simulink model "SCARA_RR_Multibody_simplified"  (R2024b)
settings: Solver=VariableStepAuto  StartTime=0.0  StopTime=5  RelTol=1e-3  EnableMultiTasking=on
undefined symbols (not defined in the file or in its folder): deg, kg, m, N, s
libraries: sm_lib x11, nesl_utility x9

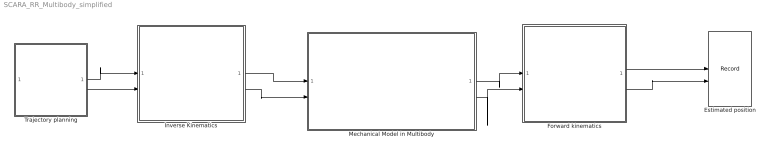
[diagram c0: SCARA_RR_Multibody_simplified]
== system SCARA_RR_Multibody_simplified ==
  Estimated position : Record  FileSettingsInternal="{\"entries\":[{\"content\":{\"excelSettings\":{\"content\":{},\"type\":\"Streamout.ExcelSettings\"}},\"type\":\"Streamout.FileSettingStorage\",\"uuid\":\"\"}],\"packageUris\":[\"http:\\/\\/schema.mathworks.com\\/mf0\\/streamout_blocks\\/R2020a\"],\"version\":\"1.0\"}"  Layout=[1 1]  SignalsInternal="{\"entries\":[{\"content\":{\"signals\":[{\"content\":{\"blockPath\":[],\"dimensions\":[1],\"domain\":\"\",\"lineColor\":\"#ff6929\",\"lineWidth\":2,\"port\":1,\"sid\":[\"\"],\"signalID\":1,\"signalName\":\"Forward kinematics:1\"},\"type\":\"RecordBlkView.Signal\",\"uuid\":\"\"},{\"content\":{\"blockPath\":[],\"dimensions\":[1],\"domain\":\"\",\"lineColor\":\"#b746ff\",\"lineWidth\":2,\"port\":2,\"sid\":[\"\"],\"signalID\":2,\"signalName\":\"Forward kinematics:2\"},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"  VisualizationBindings="{\"xyplotplugin\":{\"info\":[{\"series\":[],\"subplotID\":1}]}}"  CompatibilityTag=XY  st=-1
  Forward kinematics : MATLAB Function  TreatAsAtomicUnit=on
  Inverse Kinematics : MATLAB Function  TreatAsAtomicUnit=on
  Mechanical Model in Multibody : Subsystem
  Trajectory planning : Subsystem
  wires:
  Forward kinematics/2(Y) -> Estimated position/2
  Forward kinematics/1(X) -> Estimated position/1
  Trajectory planning/1(Xd) -> Inverse Kinematics/1(Xd)
  Trajectory planning/2(Yd) -> Inverse Kinematics/2(Yd)
  Inverse Kinematics/1(Theta1) -> Mechanical Model in Multibody/1(Theta1d)
  Inverse Kinematics/2(Theta2) -> Mechanical Model in Multibody/2(Theta 2d)
  Mechanical Model in Multibody/1(Theta1) -> Forward kinematics/1(Theta1)
  Mechanical Model in Multibody/2(Theta2) -> Forward kinematics/2(Theta2)

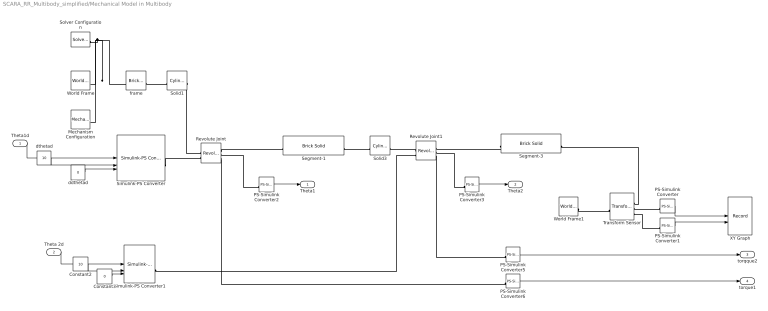
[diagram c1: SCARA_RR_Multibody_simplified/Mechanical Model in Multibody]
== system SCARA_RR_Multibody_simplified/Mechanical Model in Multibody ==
  Theta1d : Inport
  Theta 2d : Inport  Port=2
  Constant2 : Constant  Value=10
  Constant3 : Constant  Value=0
  Mechanism Configuration : sm_lib/Utilities/Mechanism Configuration  UniformGravity=Constant  GravityVector=[0 -9.80665 0]  GravityVectorUnits=m/s^2  LinearizationDelta=0.001  JointModeTransitionNonlinearIterations=2
  PS-Simulink Converter{,1..3,5..6} (6 alike) : nesl_utility/PS-Simulink Converter  PhysicalDomain=network_engine_domain  SubClassName=ps_output  LeftPortType=input  RightPortType=output  PseudoPeriodic=off  Frequencies=[]  VectorFormat=1-D array  Unit=1  AffineConversion=off
  Revolute Joint : sm_lib/Joints/Revolute Joint  JointMode=Normal  CompositeWrenchDir=FollowerOnBase  CompositeWrenchFrame=BaseFrame  SenseConstraintForce=off  SenseConstraintTorque=off  SenseTotalForce=off  SenseTotalTorque=off  PositionTargetSpecify=off  PositionTargetPriority=High  PositionTargetValue=0  PositionTargetValueUnits=deg  VelocityTargetSpecify=off  VelocityTargetPriority=High  VelocityTargetValue=0  VelocityTargetValueUnits=deg/s  EquilibriumPosition=0  EquilibriumPositionUnits=deg  SpringStiffness=0  SpringStiffnessUnits=N*m/deg  DampingCoefficient=0  DampingCoefficientUnits=N*m/(deg/s)  LowerLimitSpecify=off  LowerLimitBound=-90  LowerLimitBoundUnits=deg  LowerLimitStiffness=1e4  LowerLimitStiffnessUnits=N*m/deg  LowerLimitDamping=10  LowerLimitDampingUnits=N*m/(deg/s)  LowerLimitTransitionRegionWidth=0.1  LowerLimitTransitionRegionWidthUnits=deg  UpperLimitSpecify=off  UpperLimitBound=90  UpperLimitBoundUnits=deg  UpperLimitStiffness=1e4  UpperLimitStiffnessUnits=N*m/deg  UpperLimitDamping=10  UpperLimitDampingUnits=N*m/(deg/s)  UpperLimitTransitionRegionWidth=0.1  UpperLimitTransitionRegionWidthUnits=deg  TorqueActuationMode=ComputedTorque  MotionActuationMode=InputMotion  SensePosition=on  SenseVelocity=off  SenseAcceleration=off  SenseTorqueForce=on  SenseLowerLimitTorqueForce=off  SenseUpperLimitTorqueForce=off
  Revolute Joint1 : sm_lib/Joints/Revolute Joint  JointMode=Normal  CompositeWrenchDir=FollowerOnBase  CompositeWrenchFrame=BaseFrame  SenseConstraintForce=off  SenseConstraintTorque=off  SenseTotalForce=off  SenseTotalTorque=off  PositionTargetSpecify=off  PositionTargetPriority=High  PositionTargetValue=0  PositionTargetValueUnits=deg  VelocityTargetSpecify=off  VelocityTargetPriority=High  VelocityTargetValue=0  VelocityTargetValueUnits=deg/s  EquilibriumPosition=0  EquilibriumPositionUnits=deg  SpringStiffness=0  SpringStiffnessUnits=N*m/deg  DampingCoefficient=0  DampingCoefficientUnits=N*m/(deg/s)  LowerLimitSpecify=off  LowerLimitBound=-90  LowerLimitBoundUnits=deg  LowerLimitStiffness=1e4  LowerLimitStiffnessUnits=N*m/deg  LowerLimitDamping=10  LowerLimitDampingUnits=N*m/(deg/s)  LowerLimitTransitionRegionWidth=0.1  LowerLimitTransitionRegionWidthUnits=deg  UpperLimitSpecify=off  UpperLimitBound=90  UpperLimitBoundUnits=deg  UpperLimitStiffness=1e4  UpperLimitStiffnessUnits=N*m/deg  UpperLimitDamping=10  UpperLimitDampingUnits=N*m/(deg/s)  UpperLimitTransitionRegionWidth=0.1  UpperLimitTransitionRegionWidthUnits=deg  TorqueActuationMode=ComputedTorque  MotionActuationMode=InputMotion  SensePosition=on  SenseVelocity=off  SenseAcceleration=off  SenseTorqueForce=on  SenseLowerLimitTorqueForce=off  SenseUpperLimitTorqueForce=off
  Segment-1 : sm_lib/Body Elements/Brick Solid  BrickDimensions=[100 15 5]  BrickDimensionsUnits=cm  ExportEntireGeometry=off  InertiaType=CalculateFromGeometry  BasedOnType=Density  Density=1000  DensityUnits=kg/m^3  Mass=1  MassUnits=kg  CenterOfMass=[0 0 0]  CenterOfMassUnits=m  MomentsOfInertia=[1 1 1]  MomentsOfInertiaUnits=kg*m^2  ProductsOfInertia=[1 1 1]  ProductsOfInertiaUnits=kg*m^2  GraphicType=FromGeometry  MarkerShape=Sphere  MarkerSize=10  GraphicVisPropType=SimpleVisualProperties  GraphicDiffuseColor=[1.0 0.4 0.4]  GraphicOpacity=1.0  GraphicSpecularColor=[0.5 0.5 0.5 1.0]  GraphicAmbientColor=[0.15 0.15 0.15 1.0]  GraphicEmissiveColor=[0.0 0.0 0.0 1.0]  GraphicShininess=75  DoExposeReferenceFrame=off  SerializedFrames=<Frames><Frame><Id>Frame1</Id><Value><Name>L</Name><Origin><Source>GeometricFeature</Source><FeatureName>-x surface</FeatureName></Origin><PrimaryAxis><DefinedDirection>+Z</DefinedDirection><Source>ReferenceFrame</Source><SourceDirection>+Z</SourceDirection><FeatureName></FeatureName></PrimaryAxis><SecondaryAxis><DefinedDirection>+X</DefinedDirection><Source>ReferenceFrame</Source><SourceDirection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
  Segment-3 : sm_lib/Body Elements/Brick Solid  BrickDimensions=[100 15 5]  BrickDimensionsUnits=cm  ExportEntireGeometry=off  InertiaType=CalculateFromGeometry  BasedOnType=Density  Density=1000  DensityUnits=kg/m^3  Mass=1  MassUnits=kg  CenterOfMass=[0 0 0]  CenterOfMassUnits=m  MomentsOfInertia=[1 1 1]  MomentsOfInertiaUnits=kg*m^2  ProductsOfInertia=[1 1 1]  ProductsOfInertiaUnits=kg*m^2  GraphicType=FromGeometry  MarkerShape=Sphere  MarkerSize=10  GraphicVisPropType=SimpleVisualProperties  GraphicDiffuseColor=[0.3922 0.8314 0.07451]  GraphicOpacity=1.0  GraphicSpecularColor=[0.5 0.5 0.5 1.0]  GraphicAmbientColor=[0.15 0.15 0.15 1.0]  GraphicEmissiveColor=[0.0 0.0 0.0 1.0]  GraphicShininess=75  DoExposeReferenceFrame=off  SerializedFrames=<Frames><Frame><Id>Frame1</Id><Value><Name>L</Name><Origin><Source>GeometricFeature</Source><FeatureName>-x surface</FeatureName></Origin><PrimaryAxis><DefinedDirection>+Z</DefinedDirection><Source>ReferenceFrame</Source><SourceDirection>+Z</SourceDirection><FeatureName></FeatureName></PrimaryAxis><SecondaryAxis><DefinedDirection>+X</DefinedDirection><Source>ReferenceFrame</Source><SourceDirection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
  Simulink-PS Converter : nesl_utility/Simulink-PS Converter  PhysicalDomain=network_engine_domain  SubClassName=ps_input  LeftPortType=input  RightPortType=output  PseudoPeriodic=off  Frequencies=[]  NoiseDistribution=none  NoiseParameters=[]  Unit=1  AffineConversion=off  FilteringAndDerivatives=provide  SimscapeFilterOrder=1  InputFilterTimeConstant=0.001  UdotUserProvided=2
  Simulink-PS Converter1 : nesl_utility/Simulink-PS Converter  PhysicalDomain=network_engine_domain  SubClassName=ps_input  LeftPortType=input  RightPortType=output  PseudoPeriodic=off  Frequencies=[]  NoiseDistribution=none  NoiseParameters=[]  Unit=1  AffineConversion=off  FilteringAndDerivatives=provide  SimscapeFilterOrder=1  InputFilterTimeConstant=0.001  UdotUserProvided=2
  Solid1 : sm_lib/Body Elements/Cylindrical Solid  CylinderRadius=5  CylinderRadiusUnits=cm  CylinderLength=6  CylinderLengthUnits=cm  ExportEntireGeometry=off  InertiaType=CalculateFromGeometry  BasedOnType=Density  Density=1000  DensityUnits=kg/m^3  Mass=1  MassUnits=kg  CenterOfMass=[0 0 0]  CenterOfMassUnits=m  MomentsOfInertia=[1 1 1]  MomentsOfInertiaUnits=kg*m^2  ProductsOfInertia=[1 1 1]  ProductsOfInertiaUnits=kg*m^2  GraphicType=FromGeometry  MarkerShape=Sphere  MarkerSize=10  GraphicVisPropType=SimpleVisualProperties  GraphicDiffuseColor=[0.8 0.0 0.0]  GraphicOpacity=1.0  GraphicSpecularColor=[0.5 0.5 0.5 1.0]  GraphicAmbientColor=[0.15 0.15 0.15 1.0]  GraphicEmissiveColor=[0.0 0.0 0.0 1.0]  GraphicShininess=75  DoExposeReferenceFrame=off  SerializedFrames=<Frames><Frame><Id>Frame1</Id><Value><Name>L</Name><Origin><Source>GeometricFeature</Source><FeatureName>top surface</FeatureName></Origin><PrimaryAxis><DefinedDirection>+Z</DefinedDirection><Source>ReferenceFrame</Source><SourceDirection>+Z</SourceDirection><FeatureName></FeatureName></PrimaryAxis><SecondaryAxis><DefinedDirection>+X</DefinedDirection><Source>ReferenceFrame</Source><SourceDirectio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
  Solid3 : sm_lib/Body Elements/Cylindrical Solid  CylinderRadius=5  CylinderRadiusUnits=cm  CylinderLength=6  CylinderLengthUnits=cm  ExportEntireGeometry=off  InertiaType=CalculateFromGeometry  BasedOnType=Density  Density=1000  DensityUnits=kg/m^3  Mass=1  MassUnits=kg  CenterOfMass=[0 0 0]  CenterOfMassUnits=m  MomentsOfInertia=[1 1 1]  MomentsOfInertiaUnits=kg*m^2  ProductsOfInertia=[1 1 1]  ProductsOfInertiaUnits=kg*m^2  GraphicType=FromGeometry  MarkerShape=Sphere  MarkerSize=10  GraphicVisPropType=SimpleVisualProperties  GraphicDiffuseColor=[0.8 0.0 0.0]  GraphicOpacity=1.0  GraphicSpecularColor=[0.5 0.5 0.5 1.0]  GraphicAmbientColor=[0.15 0.15 0.15 1.0]  GraphicEmissiveColor=[0.0 0.0 0.0 1.0]  GraphicShininess=75  DoExposeReferenceFrame=off  SerializedFrames=<Frames><Frame><Id>Frame1</Id><Value><Name>L</Name><Origin><Source>GeometricFeature</Source><FeatureName>top surface</FeatureName></Origin><PrimaryAxis><DefinedDirection>+Z</DefinedDirection><Source>ReferenceFrame</Source><SourceDirection>+Z</SourceDirection><FeatureName></FeatureName></PrimaryAxis><SecondaryAxis><DefinedDirection>+X</DefinedDirection><Source>ReferenceFrame</Source><SourceDirectio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
  Solver Configuration : nesl_utility/Solver Configuration  PhysicalDomain=network_engine_domain  SubClassName=solver  LeftPortType=input  RightPortType=generic  Tones=[]  Harmonics=[]  SimulateNoise=off  Profile=off  UseLocalSampling=off  EnableSwitchedLinearOptims=on  FrequencyDomain=off  UseCCode=off  RelTol=0.001  AbsTol=1e-06  MinStep=1e-09  ToWorkspace=off  RevertToSquareIcSolve=off  NumHomotopyIterations=100  PhasorMode=off  PhasorModeNumHarmonics=1  ConsistencySolver=NEWTON_FTOL  IndexReductionMethod=DerivativeReplacement  DoDC=off  ResidualTolerance=1e-09  ConsistencyTolSource=GLOBAL  ConsistencyAbsTol=0.001  ConsistencyRelTol=0.001  ConsistencyTolFactor=0.001  UseLocalSolver=off  LocalSolverChoice=NE_BACKWARD_EULER_ADVANCER  ResolveIndetEquations=on  FunctionEvalNumThread=1  LocalSolverSampleTime=0.001  DoFixedCost=off  MaxNonlinIter=3  MaxModeIter=2  ComputeImpulses=off  ImpulseIterations=2  LinearAlgebra=Sparse  LinearAlgebraNumThread=0  EquationFormulation=NE_TIME_EF  DelaysMemoryBudget=1024  AutomaticFiltering=on  FilteringTimeConstant=0.001  PartitionStorageMethod=AS_NEEDED  PartitionMemoryBudget=1024  PartitionMethod=FAST  MultibodyUseLocalSolver=off  MultibodyLocalSolverChoice=ODE1  MultibodyLocalSolverSampleTime=0.001
  Transform Sensor : sm_lib/Frames and Transforms/Transform Sensor  MeasurementFrame=World  RotationSequence=XYX  SenseAngle=off  SenseAxis=off  SenseQ=off  SenseR=off  SenseRotationSequence=off  SenseOmegaX=off  SenseOmegaY=off  SenseOmegaZ=off  SenseOmega=off  SenseQDot=off  SenseRDot=off  SenseRotationSequenceDot=off  SenseAlphaX=off  SenseAlphaY=off  SenseAlphaZ=off  SenseAlpha=off  SenseQDDot=off  SenseRDDot=off  SenseX=on  SenseY=on  SenseZ=off  SenseXYZ=off  SenseRad=off  SenseAzim=off  SenseDist=off  SenseInc=off  SenseXDot=off  SenseYDot=off  SenseZDot=off  SenseXYZDot=off  SenseRadDot=off  SenseAzimDot=off  SenseDistDot=off  SenseIncDot=off  SenseXDDot=off  SenseYDDot=off  SenseZDDot=off  SenseXYZDDot=off  SenseRadDDot=off  SenseAzimDDot=off  SenseDistDDot=off  SenseIncDDot=off
  World Frame : sm_lib/Frames and Transforms/World Frame
  World Frame1 : sm_lib/Frames and Transforms/World Frame
  XY Graph : Record  FileSettingsInternal="{\"entries\":[{\"content\":{\"excelSettings\":{\"content\":{},\"type\":\"Streamout.ExcelSettings\"}},\"type\":\"Streamout.FileSettingStorage\",\"uuid\":\"\"}],\"packageUris\":[\"http:\\/\\/schema.mathworks.com\\/mf0\\/streamout_blocks\\/R2020a\"],\"version\":\"1.0\"}"  Layout=[1 1]  SignalsInternal="{\"entries\":[{\"content\":{\"signals\":[{\"content\":{\"blockPath\":[],\"dimensions\":[1],\"domain\":\"\",\"lineColor\":\"#a2142f\",\"plots\":[ 1 ],\"port\":1,\"sid\":[\"\"],\"signalID\":1,\"signalName\":\"PS-Simulink\\nConverter\"},\"type\":\"RecordBlkView.Signal\",\"uuid\":\"\"},{\"content\":{\"blockPath\":[],\"dimensions\":[1],\"domain\":\"\",\"lineColor\":\"#139fff\",\"plots\":[ 1 ],\"port\":2,\"sid\":[\"\"],\"signalID\":2,\"signalName\":\"PS-Simulink\\nConverte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"  VisualizationBindings="{\"xyplotplugin\":{\"info\":[{\"series\":[{\"bindingParametersList\":[{\"parameter\":\"X-Axis\",\"signalID\":1,\"signalName\":\"PS-Simulink\\nConverter\"},{\"parameter\":\"Y-Axis\",\"signalID\":2,\"signalName\":\"PS-Simulink\\nConverter1\"}],\"seriesID\":0}],\"subplotID\":1}]}}"  CompatibilityTag=XY  st=-1
  ddthetad : Constant  Value=0
  dthetad : Constant  Value=10
  frame : sm_lib/Body Elements/Brick Solid  BrickDimensions=[15 15 5]  BrickDimensionsUnits=cm  ExportEntireGeometry=off  InertiaType=CalculateFromGeometry  BasedOnType=Density  Density=1000  DensityUnits=kg/m^3  Mass=1  MassUnits=kg  CenterOfMass=[0 0 0]  CenterOfMassUnits=m  MomentsOfInertia=[1 1 1]  MomentsOfInertiaUnits=kg*m^2  ProductsOfInertia=[1 1 1]  ProductsOfInertiaUnits=kg*m^2  GraphicType=FromGeometry  MarkerShape=Sphere  MarkerSize=10  GraphicVisPropType=SimpleVisualProperties  GraphicDiffuseColor=[0.0 0.0 0.6]  GraphicOpacity=1.0  GraphicSpecularColor=[0.5 0.5 0.5 1.0]  GraphicAmbientColor=[0.15 0.15 0.15 1.0]  GraphicEmissiveColor=[0.0 0.0 0.0 1.0]  GraphicShininess=75  DoExposeReferenceFrame=on  SerializedFrames=<Frames><Frame><Id>Frame1</Id><Value><Name>F</Name><Origin><Source>GeometricFeature</Source><FeatureName>-z surface</FeatureName></Origin><PrimaryAxis><DefinedDirection>+Z</DefinedDirection><Source>ReferenceFrame</Source><SourceDirection>+Z</SourceDirection><FeatureName></FeatureName></PrimaryAxis><SecondaryAxis><DefinedDirection>+X</DefinedDirection><Source>ReferenceFrame</Source><SourceDirection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
  Theta1 : Outport  VectorParamsAs1DForOutWhenUnconnected=off
  Theta2 : Outport  Port=2  VectorParamsAs1DForOutWhenUnconnected=off
  torqque2 : Outport  Port=3  VectorParamsAs1DForOutWhenUnconnected=off
  torque1 : Outport  Port=4  VectorParamsAs1DForOutWhenUnconnected=off
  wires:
  PS-Simulink Converter/1 -> XY Graph/1
  dthetad/1 -> Simulink-PS Converter/2
  Theta 2d/1 -> Simulink-PS Converter1/1
  PS-Simulink Converter1/1 -> XY Graph/2
  Theta1d/1 -> Simulink-PS Converter/1
  ddthetad/1 -> Simulink-PS Converter/3
  PS-Simulink Converter2/1 -> Theta1/1
  Constant3/1 -> Simulink-PS Converter1/3
  Constant2/1 -> Simulink-PS Converter1/2
  PS-Simulink Converter3/1 -> Theta2/1
  PS-Simulink Converter5/1 -> torqque2/1
  PS-Simulink Converter6/1 -> torque1/1
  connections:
  Segment-3/LConn1 -- Revolute Joint1/RConn1
  Revolute Joint1/LConn1 -- Solid3/RConn1
  PS-Simulink Converter3/LConn1 -- Revolute Joint1/RConn2
  PS-Simulink Converter/LConn1 -- Transform Sensor/RConn2
  Transform Sensor/RConn3 -- PS-Simulink Converter1/LConn1
  Solver Configuration/RConn1 -- Mechanism Configuration/RConn1 -- frame/RConn1 -- World Frame/RConn1
  Simulink-PS Converter1/RConn1 -- Revolute Joint1/LConn2
  PS-Simulink Converter2/LConn1 -- Revolute Joint/RConn2
  Revolute Joint/RConn1 -- Segment-1/LConn1
  Solid3/LConn1 -- Segment-1/RConn1
  World Frame1/RConn1 -- Transform Sensor/LConn1
  Transform Sensor/RConn1 -- Segment-3/RConn1
  frame/LConn1 -- Solid1/LConn1
  Simulink-PS Converter/RConn1 -- Revolute Joint/LConn2
  Solid1/RConn1 -- Revolute Joint/LConn1
  Revolute Joint/RConn3 -- PS-Simulink Converter6/LConn1
  Revolute Joint1/RConn3 -- PS-Simulink Converter5/LConn1

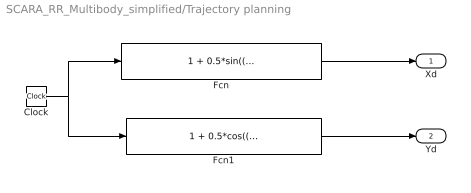
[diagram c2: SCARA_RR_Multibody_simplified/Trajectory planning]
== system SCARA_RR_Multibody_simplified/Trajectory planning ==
  Clock : Clock
  Fcn : Fcn  Expr=1 + 0.5*sin((2*pi/5)*u + pi/2)
  Fcn1 : Fcn  Expr=1 + 0.5*cos((2*pi/5)*u + pi/2)
  Xd : Outport  VectorParamsAs1DForOutWhenUnconnected=off
  Yd : Outport  Port=2  VectorParamsAs1DForOutWhenUnconnected=off
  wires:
  Clock/1 -> Fcn1/1, Fcn/1
  Fcn/1 -> Xd/1
  Fcn1/1 -> Yd/1

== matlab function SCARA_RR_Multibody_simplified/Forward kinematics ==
function [X,Y] = Forwardkinematics(Theta1,Theta2)

l1 = 1; %Chieu dai cua link 1 l1 = 1(m)
l2 = 1;

T10 = [cos(Theta1), -sin(Theta1), 0, l1*cos(Theta1);
       sin(Theta1), cos(Theta1),  0, l1*sin(Theta1);
       0,          0,             1,      0;
       0,          0,             0,       1];

T21 = [cos(Theta2), -sin(Theta2), 0, l2*cos(Theta2);
       sin(Theta2), cos(Theta2),  0, l2*sin(Theta2);
       0,          0,             1,      0;
       0,          0,             0,       1];

T20 = T10*T21;

X = T20(1,4);
Y = T20(2,4);

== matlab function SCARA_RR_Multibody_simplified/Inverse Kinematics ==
function [Theta1,Theta2] = InverseKinematics(Xd,Yd)

l1 = 1;
l2 = 1;

Theta2 = acos((Xd^2 + Yd^2 -l1^2 - l2^2)/(2*l1*l2));

s_Theta2 = sin(Theta2);
c_Theta2 = cos(Theta2);

Theta1 = atan2(Yd,Xd) - atan2(l2*s_Theta2,(l1+l2*c_Theta2));
